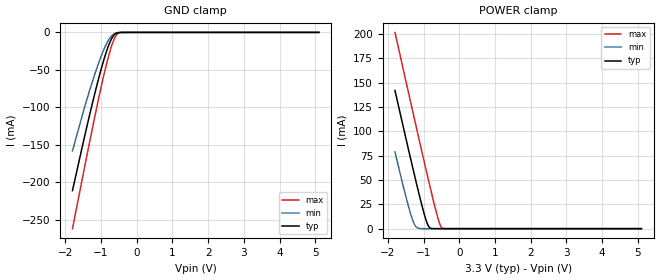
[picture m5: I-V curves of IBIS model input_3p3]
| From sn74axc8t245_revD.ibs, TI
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|   input_3p3 Model
[Model]   input_3p3
Model_type   Input
Vinl = 0.8
Vinh = 2.3
|   typ   min   max
C_comp   1.86062E-12   1.26954E-12   2.13619E-12
| Where Nom  PVT is Nominal Process, 3.3V, 27C
|   Fast PVT is Strong Process,  3.6V, -40C
|   Slow PVT is Weak Process,   3.0V, 130C
[Voltage Range]   3.3   3   3.6
|Junction Temperature
[Temperature Range]   27   130   -40
[Power Clamp Reference]   3.3   3   3.6
[GND Clamp Reference]   0   0   0
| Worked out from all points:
|   GND clamp passes 1 mA (typ) near -0.57 V on its own axis
|   POWER clamp passes 1 mA (typ) near -0.83 V on its own axis
[GND Clamp]
|   Voltage   I(typ)   I(min)   I(max)
-1.8V     -210.9mA   -157.9mA   -261.6mA
-1.49V    -144.7mA   -104.6mA   -186.5mA
-1.296V   -105.2mA   -73.69mA   -140.6mA
-1.117V   -70.54mA   -47.4mA    -99.2mA
-951.3mV  -41.37mA   -26.15mA   -63.06mA
-820.2mV  -21.52mA   -12.61mA   -37.23mA
-716.7mV  -9.415mA   -5.207mA   -19.86mA
-613.2mV  -2.39mA    -1.422mA   -6.892mA
-523.5mV  -394uA     -320.5uA   -1.365mA
-426.9mV  -33.77uA   -44.18uA   -102.3uA
-68.1mV   0A         0A         0A
5.1V      0A         0A         0A
[POWER Clamp]
|   Voltage   I(typ)   I(min)   I(max)
-1.8V     141.9mA    78.74mA    201.4mA
-1.414V   79.93mA    21.78mA    138.3mA
-1.296V   61.5mA     8.016mA    119.2mA
-1.234V   51.89mA    3.123mA    109.2mA
-1.151V   39.29mA    456.6uA    95.81mA
-985.8mV  15.65mA    4.189uA    69.3mA
-868.5mV  3.093mA    131.9nA    50.79mA
-799.5mV  400.9uA    7.757nA    40.08mA
-571.8mV  47.54nA    0A         7.669mA
-516.6mV  0A         0A         2.383mA
-468.3mV  0A         0A         390.4uA
5.1V      0A         0A         0A
